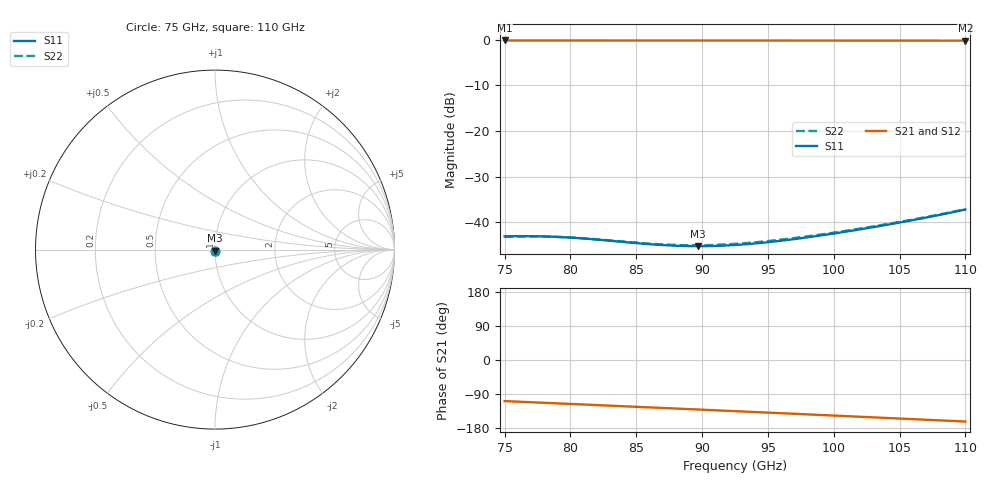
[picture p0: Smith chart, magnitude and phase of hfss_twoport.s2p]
! Touchstone file from project gndCpw
! Exported from HFSS 14.0.0
! Variables:
!  airbox_h = 500um
!  cc_h = 6.7um
!  cc_l = 2mm
!  cc_w = 70um
!  cpw_pitch = 155um
!  gap = 70um
!  l_2_via1 = 250um
!  length = 500um
!  oc_w = 70um
!  s = 30um
!  sub_h = 100um
!  sub_w = 465um
!  via_r = 30um
!  wp_w_factor = 1.3
!Data is not renormalized
# GHZ S MA
! Modal data exported
! Port[1] = 1:1
! Port[2] = 2:1
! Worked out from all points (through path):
!   101 points, 75 GHz to 110 GHz, reference per port
!   highest |S21| = -0.14 dB at 75 GHz (marker M1); lowest = -0.2 dB at 110 GHz (marker M2)
!   group delay of S21, straight-line fit = 4.28 ps
!   lowest |S11| = -45.2 dB at 89.7 GHz (marker M3), VSWR 1.01
!   |S11| at or under -10 dB: start of sweep to end of sweep
!   |S22| runs from -45.0 to -37.1 dB; largest |S21 - S12| = 5e-12
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75  0.007046 -86.2  0.9841 -108.4  0.9841 -108.4  0.006948 -85.9
! Gamma ! 10.3322101252995 3736.34654552359 9.8996147444026 3736.11167025233
! Port Impedance 49.6880494439638 -0.112098324722594 49.626538212863 -0.112974315275203
76.75  0.007081 -90.7  0.9839 -111.1  0.9839 -111.1  0.007029 -90.5
78.15  0.007024 -94.2  0.9838 -113.2  0.9838 -113.2  0.007005 -94.1
79.55  0.006887 -97.4  0.9837 -115.3  0.9837 -115.3  0.006897 -97.5
80.95  0.006683 -100.1  0.9836 -117.4  0.9836 -117.4  0.006713 -100.3
83.75  0.006167 -103.2  0.9833 -121.6  0.9833 -121.6  0.006226 -103.5
85.5  0.005859 -103.1  0.9832 -124.3  0.9832 -124.3  0.005936 -103.6
86.9  0.005667 -102.1  0.9831 -126.4  0.9831 -126.4  0.00576 -102.6
88.3  0.005544 -100.3  0.9829 -128.5  0.9829 -128.5  0.005655 -101.0
89.7  0.005502 -98.0  0.9828 -130.7  0.9828 -130.7  0.005631 -98.9
91.1  0.005544 -95.5  0.9826 -132.8  0.9826 -132.8  0.005689 -96.6
92.5  0.005669 -93.0  0.9825 -135.0  0.9825 -135.0  0.005826 -94.3
93.9  0.005872 -90.6  0.9823 -137.1  0.9823 -137.1  0.006039 -92.1
95.3  0.006148 -88.6  0.9822 -139.3  0.9822 -139.3  0.00632 -90.3
96.7  0.006492 -86.8  0.982 -141.5  0.982 -141.5  0.006667 -88.8
98.45  0.007016 -85.2  0.9817 -144.2  0.9817 -144.2  0.007191 -87.3
101.25  0.008072 -83.7  0.9813 -148.6  0.9813 -148.6  0.00824 -86.0
103  0.008884 -83.4  0.981 -151.3  0.981 -151.3  0.009046 -85.7
104.4  0.009631 -83.4  0.9808 -153.6  0.9808 -153.6  0.009787 -85.8
107.2  0.01145 -84.5  0.9803 -158.0  0.9803 -158.0  0.0116 -86.7
108.6  0.01257 -85.4  0.9799 -160.2  0.9799 -160.2  0.01271 -87.6
110  0.01386 -86.7  0.9796 -162.5  0.9796 -162.5  0.014 -88.8
